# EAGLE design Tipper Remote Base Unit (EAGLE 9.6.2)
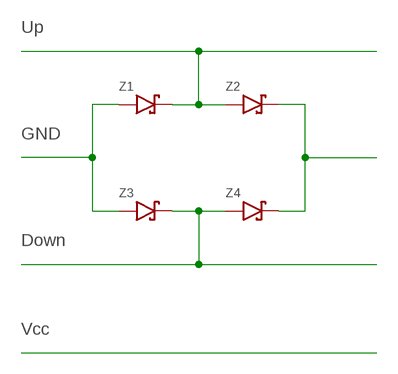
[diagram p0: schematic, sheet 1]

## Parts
Z1  DIODE-SCHOTTKY-1N5822  [DIODE_SMB]
Z2  DIODE-SCHOTTKY-1N5822  [DIODE_SMB]
Z3  DIODE-SCHOTTKY-1N5822  [DIODE_SMB]
Z4  DIODE-SCHOTTKY-1N5822  [DIODE_SMB]

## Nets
N$1: Z1.C Z2.A
N$2: Z3.C Z4.A
N$3: Z1.A Z3.A
N$4: Z2.C Z4.C

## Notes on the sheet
- Up
- GND
- Down
- Vcc

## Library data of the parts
Z1-Z4 = digitalconcepts:DIODE-SCHOTTKY-1N5822: 1N5822 Schottky Diode SMB

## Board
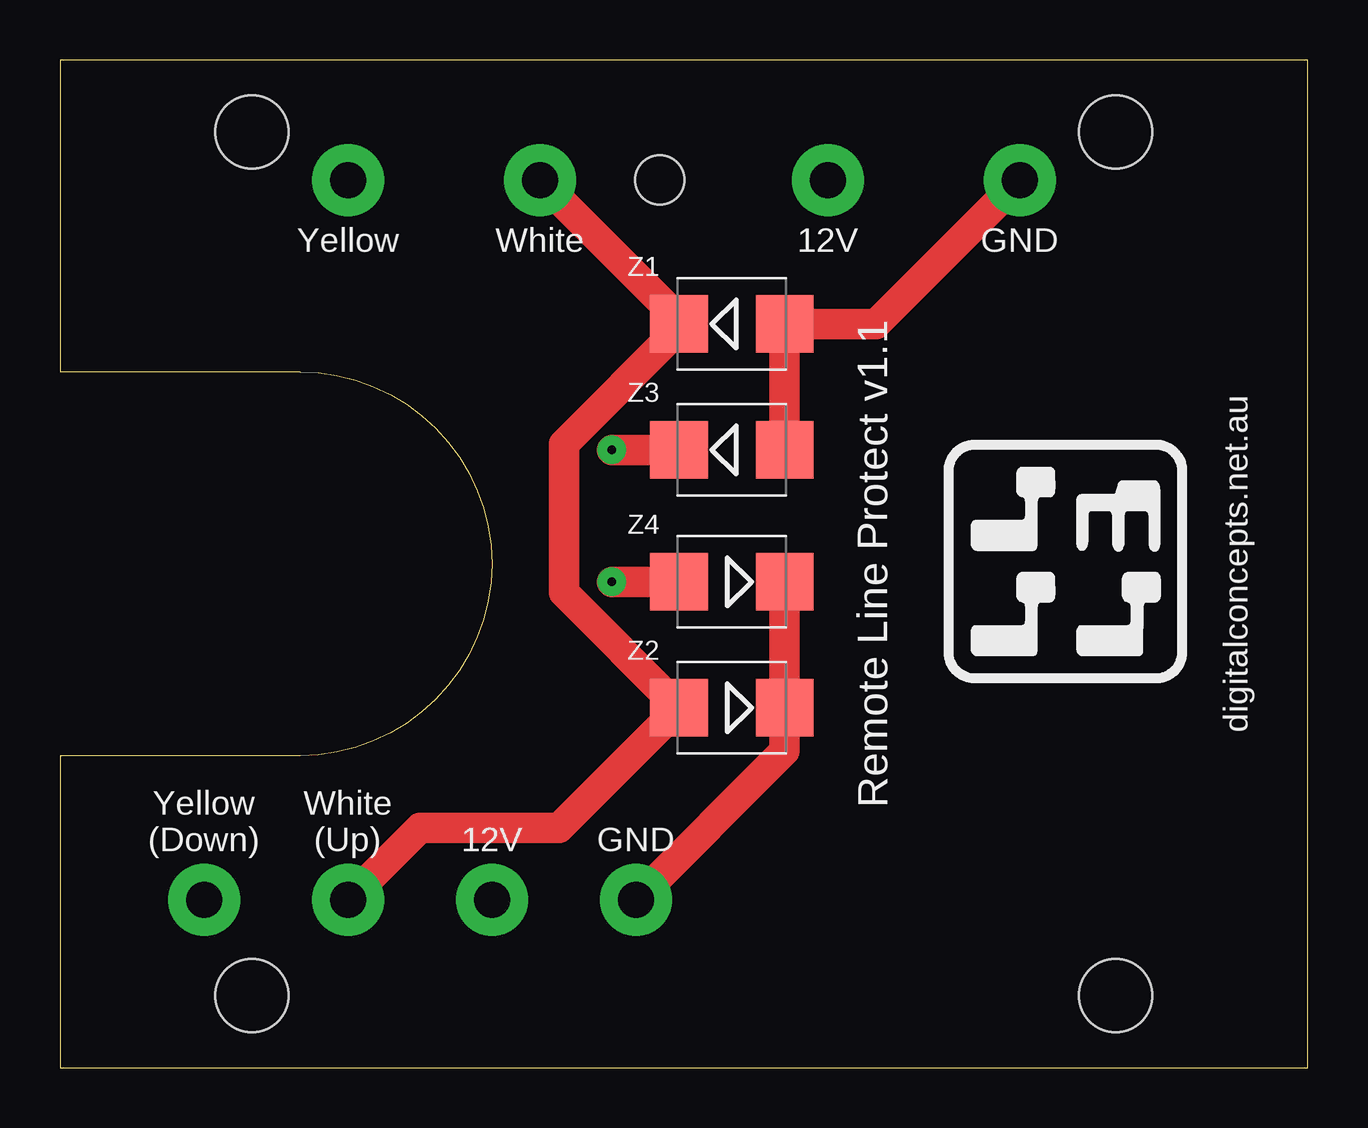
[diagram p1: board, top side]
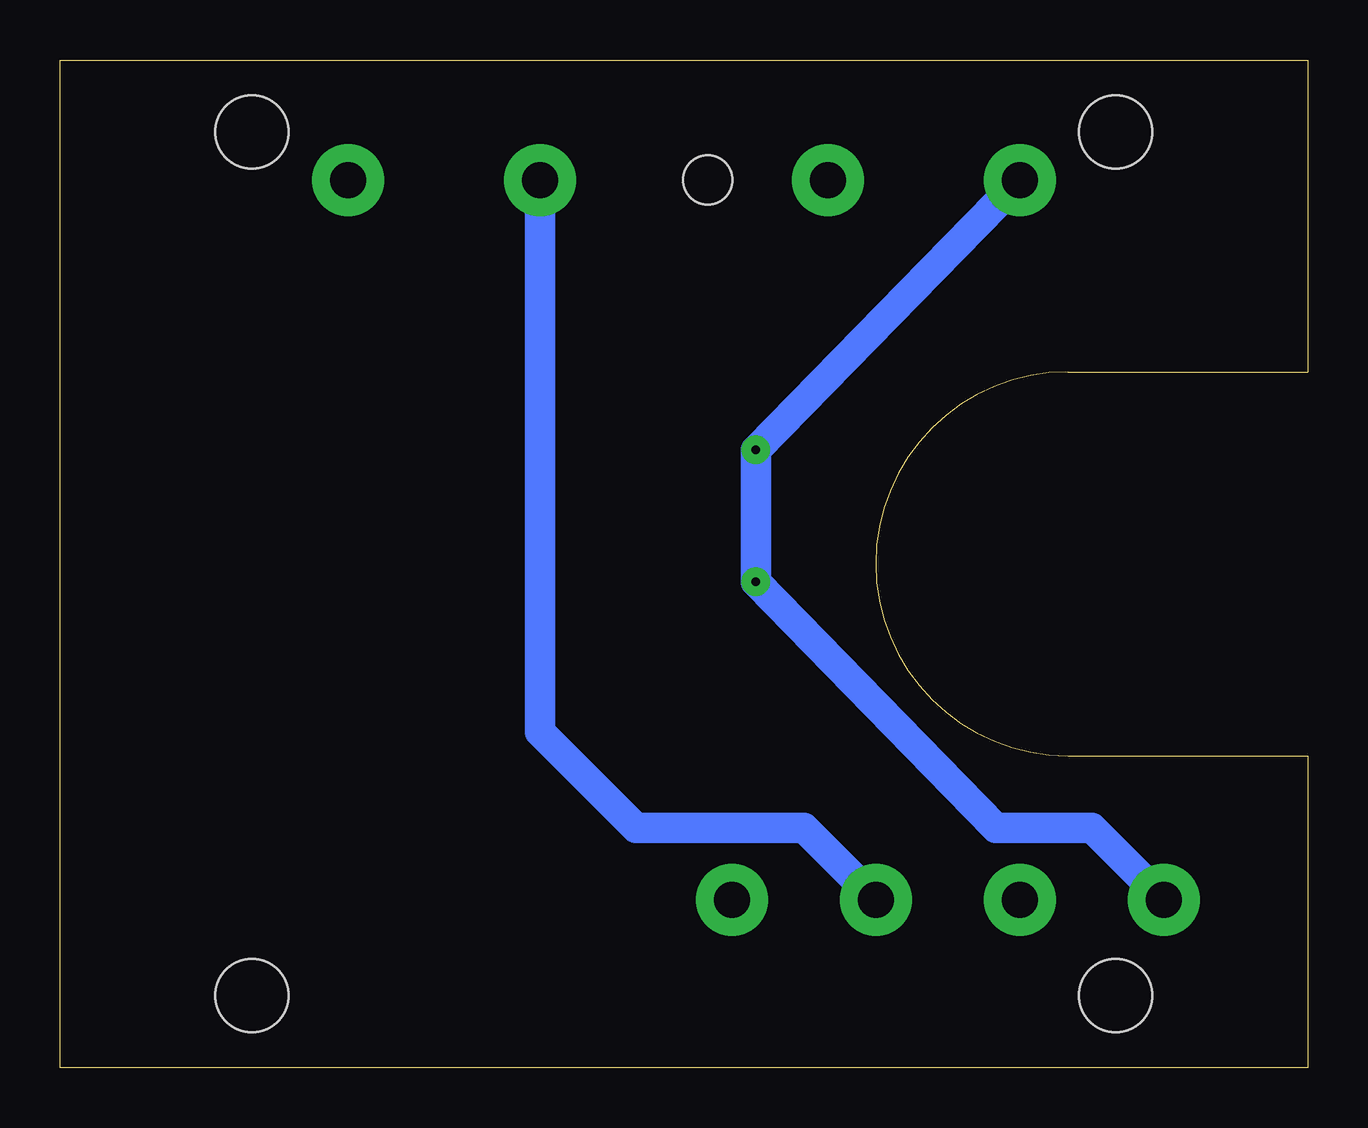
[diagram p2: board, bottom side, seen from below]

Size 52 x 42 mm. Coordinates in mm from the lower left corner, seen from the top.
Outline: 0,0 52,0 52,42 0,42 0,29 10,29 arc-180 10,13 0,13 0,0
Copper layers (1*16): Top 0.035mm / dielectric 1.5mm / Bottom 0.035mm
Design rules "default": minimum track width 6mil, minimum drill 0.35mm, track to track 6mil, track to pad 6mil, pad to pad 6mil, via to via 6mil, smd to smd 6mil, copper to edge 40mil, drill to drill 6mil, minimum pad ring 10mil, minimum via ring 8mil, stop-mask expansion 4mil, vias tented up to drill 0mil, thermal gap 10mil
Holes 2.03 mm at 25,37
Holes 3.05 mm at 44,39 44,3 8,3 8,39

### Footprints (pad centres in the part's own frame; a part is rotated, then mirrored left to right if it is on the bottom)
DIODE_SMB = smd 2.4 x 2.4: A 2.2,0; C -2.2,0

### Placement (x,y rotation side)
Z1  28,31 0 top
Z2  28,15 180 top
Z3  28,25.75 0 top
Z4  28,20.25 180 top

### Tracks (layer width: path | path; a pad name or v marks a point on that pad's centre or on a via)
N$1  (via drill 1.5 pad 3)
  Top 0.813: Z1.C 25.8,31.2
  Top 1.27: Z1.C 25.8,30.8 21,26 21,19.8 Z2.A 20.8,10 15,10 v12,7 | 25.8,31.2 v20,37
N$2  (via drill 0.35 pad 1.2, 1.5 pad 3)
  Top 1.27: Z4.A v23,20.25 | Z3.C v23,25.75
  Bottom 1.27: v6,7 9,10 13,10 v23,20.25 v23,25.75 v12,37
N$3  (via drill 1.5 pad 3)
  Top 1.27: Z3.A Z1.A 34,31 v40,37
N$4  (via drill 1.5 pad 3)
  Top 1.27: Z4.C Z2.C 30.2,13.2 v24,7
N$6  (via drill 1.5 pad 3)
  Bottom 1.27: v32,37 32,14 28,10 21,10 v18,7

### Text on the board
tPlace: Remote Line Protect v1.1 | digitalconcepts.net.au
tNames: Yellow | White | 12V | GND | Yellow / (Down) | White / (Up) | 12V | GND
